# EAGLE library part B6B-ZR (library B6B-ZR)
JST-ZH Connector 6 pol, 1.5mm pitch Package: B6B-ZR Source: http://www.jst-mfg.com/product/pdf/eng/eZH.pdf
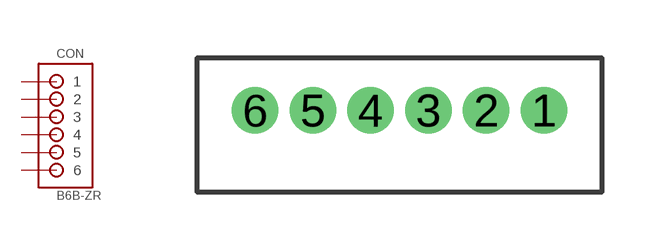
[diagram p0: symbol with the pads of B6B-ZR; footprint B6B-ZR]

Designator prefix CON

## B6B-ZR (Availability: Unavailable; Description: Connector Header Surface Mount 6 position 0.059 _1.50mm_; MF: JST; MP: B6B-ZR; Package: None; Price: None)  [B6B-ZR]
1  1
2  2
3  3
4  4
5  5
6  6

## Footprint B6B-ZR (pad centres in mm)
drill 0.7: 1 9,-1.3; 2 7.5,-1.3; 3 6,-1.3; 4 4.5,-1.3; 5 3,-1.3; 6 1.5,-1.3

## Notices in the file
This work is licensed under a Creative Commons Attribution-ShareAlike 4.0 International License (CC BY-SA) with Design Exception 1.0
